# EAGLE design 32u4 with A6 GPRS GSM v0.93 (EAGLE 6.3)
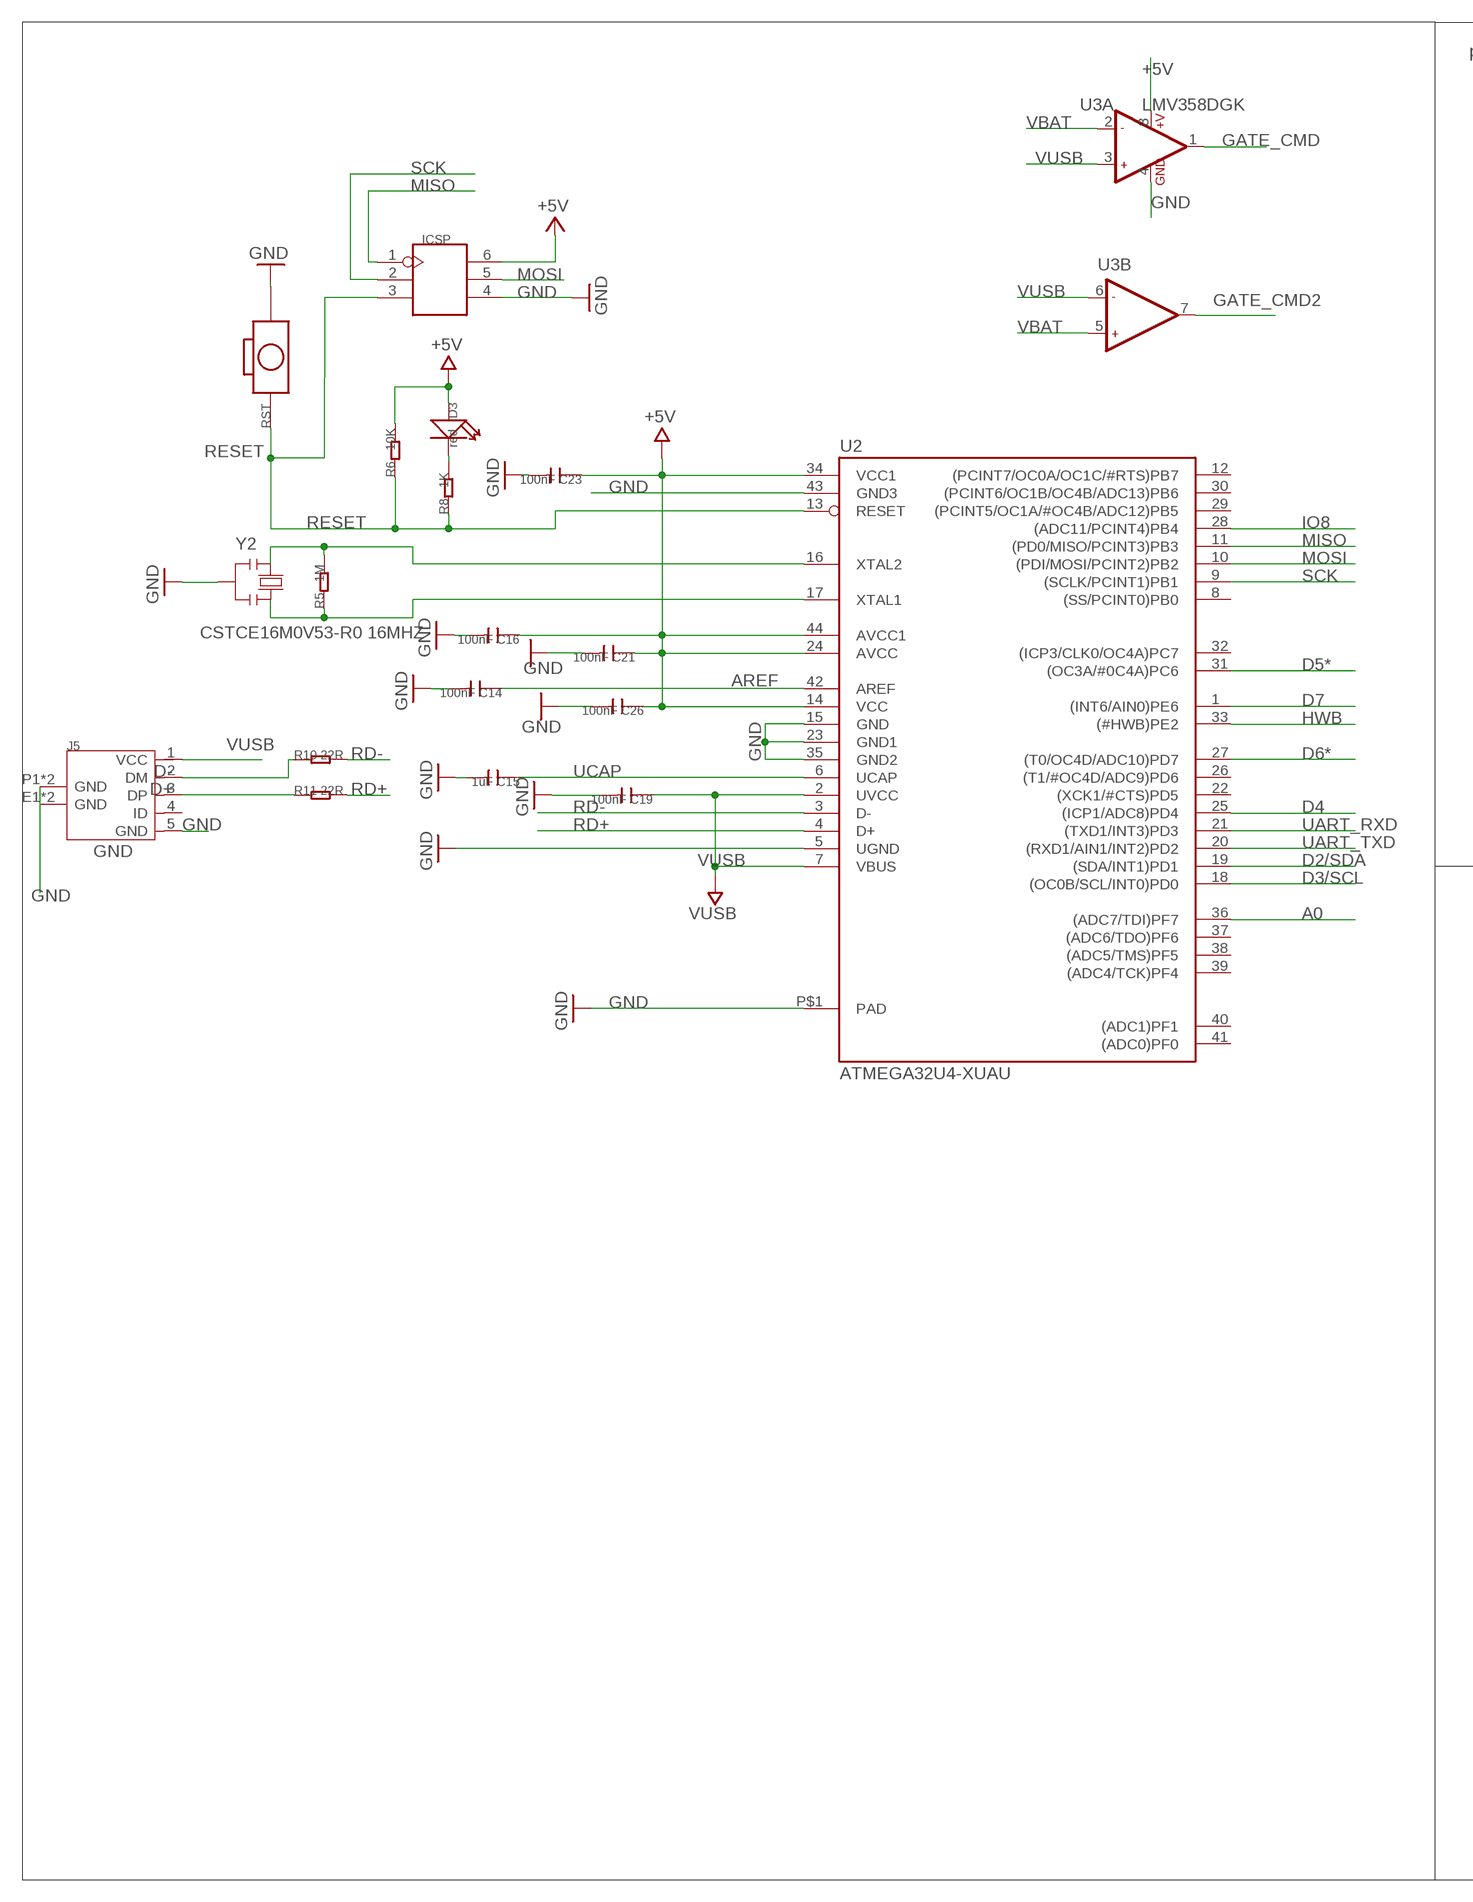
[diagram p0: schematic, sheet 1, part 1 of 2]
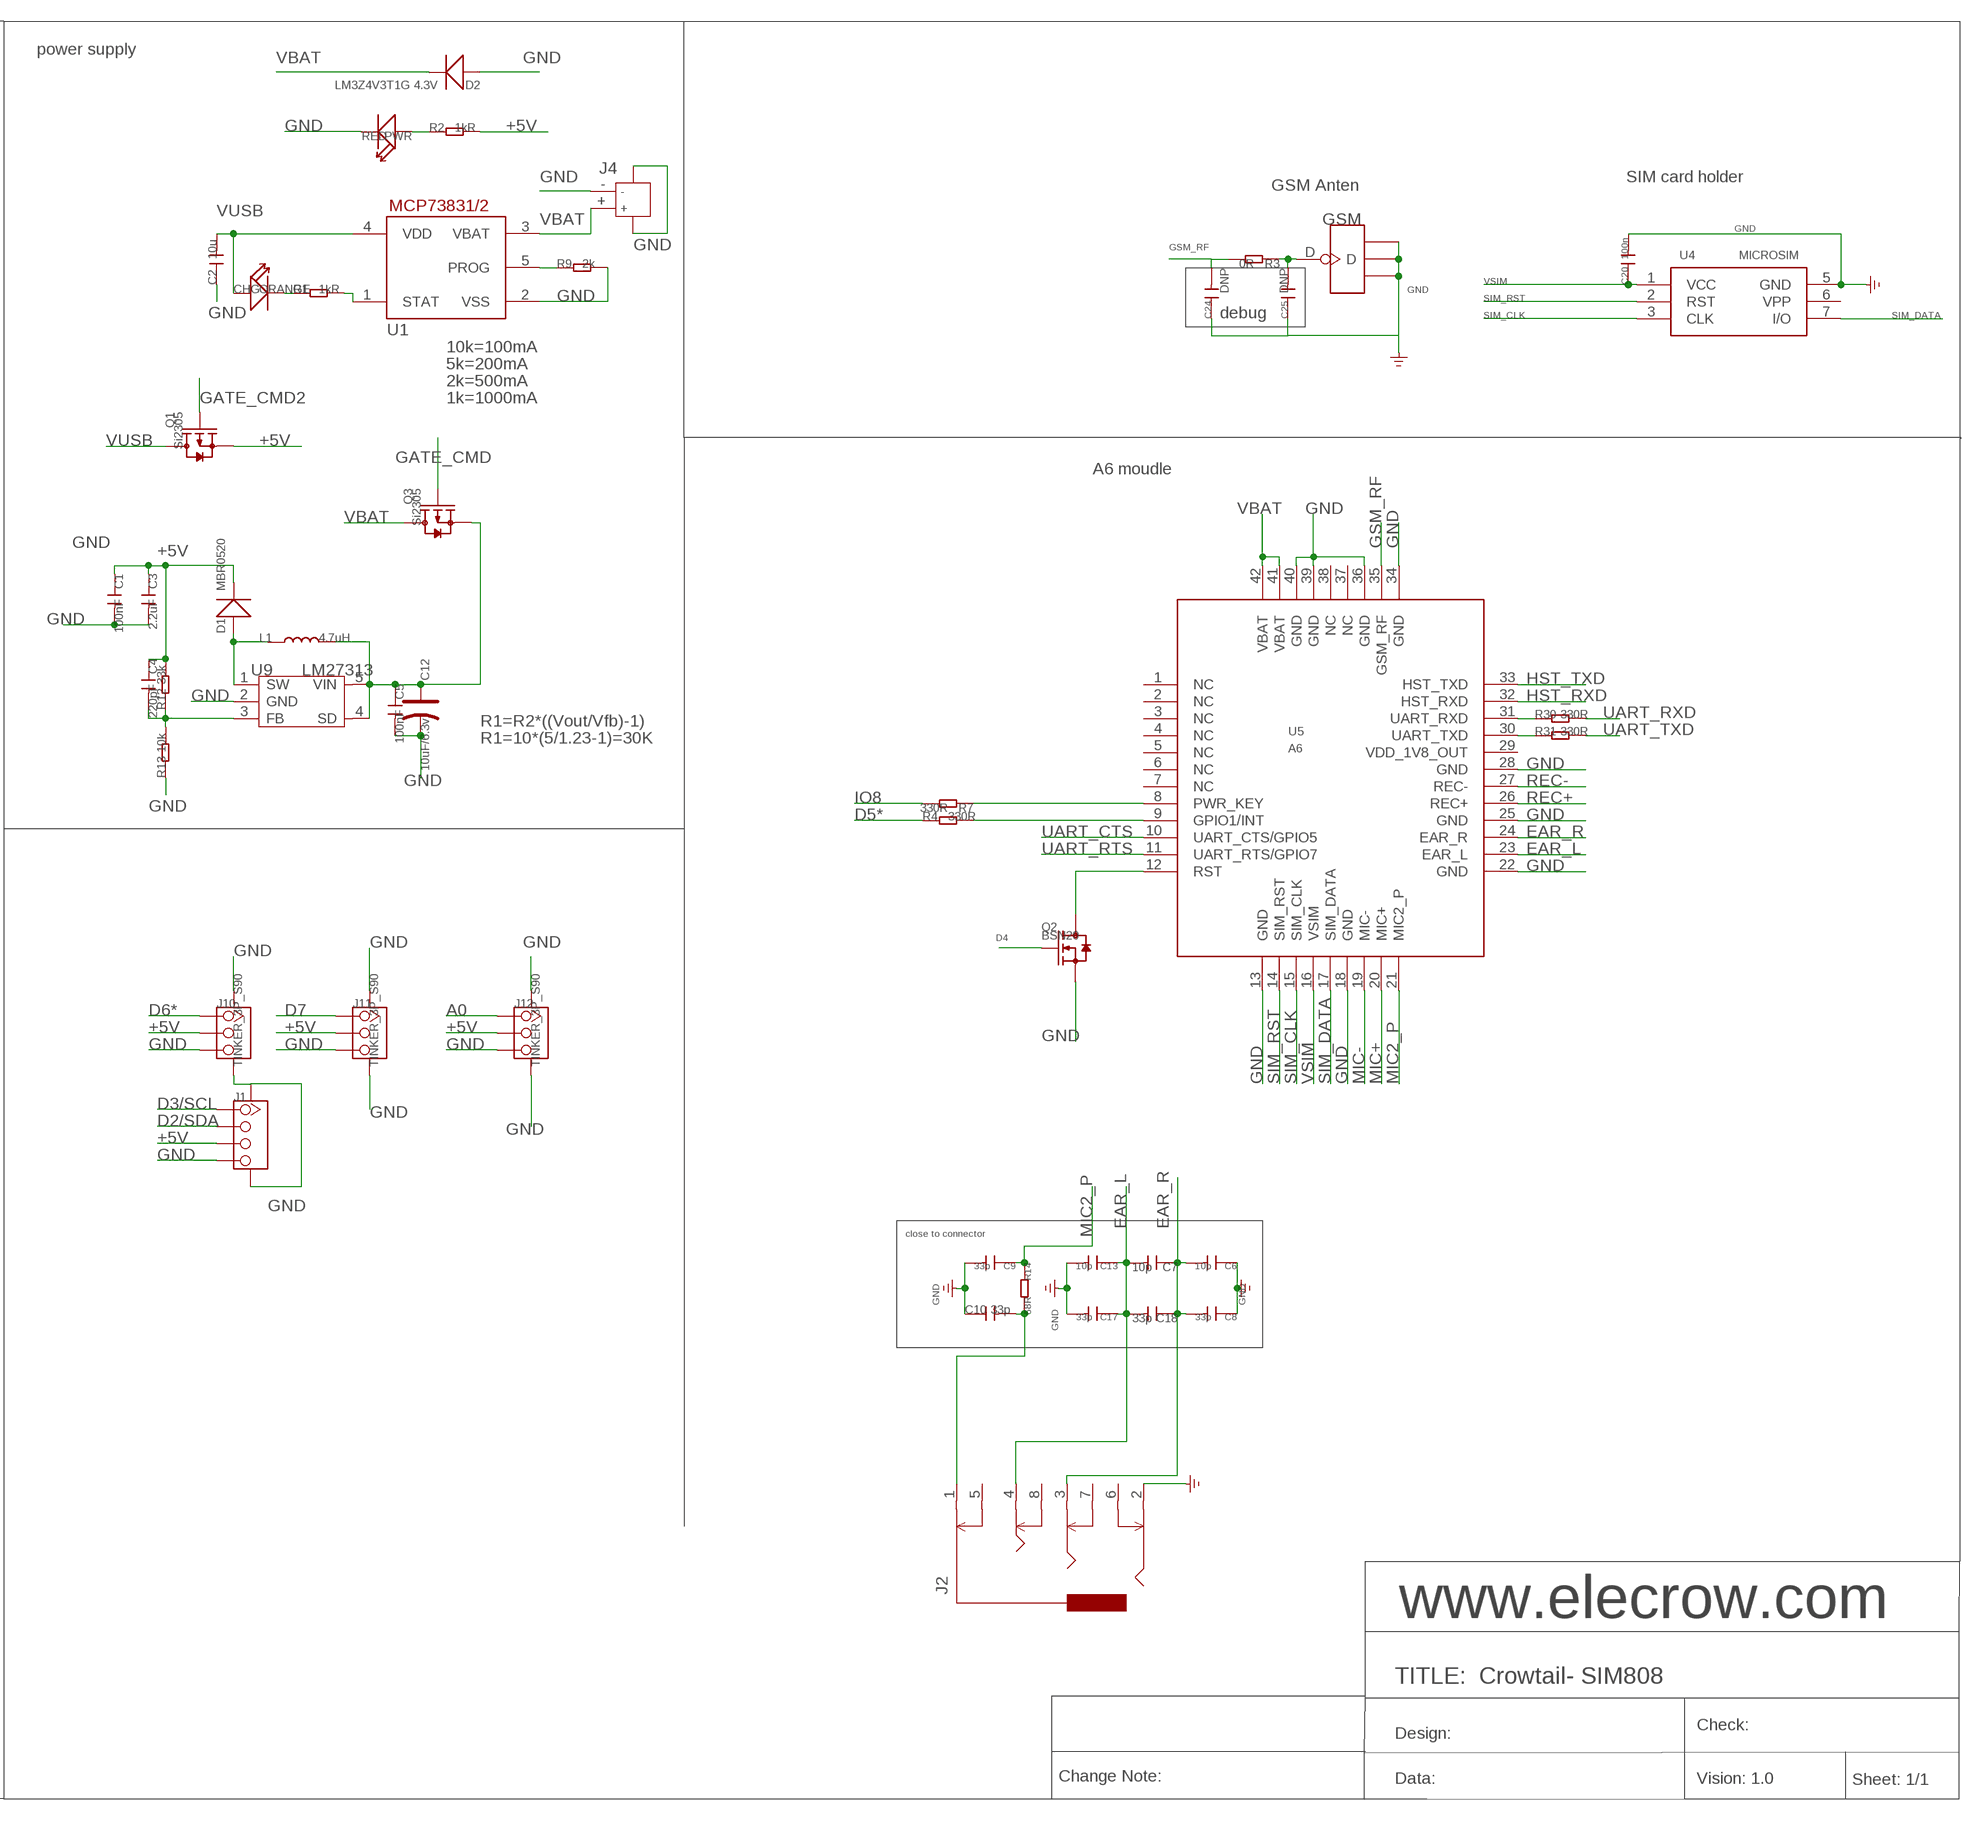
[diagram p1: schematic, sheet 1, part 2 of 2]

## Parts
C1  100nF  C-0603  [C0603]
C2  10u  C-0603  [C0603]
C3  2.2uF  C-0603  [C0603]
C4  220pF  C-0603  [C0603]
C5  100nF  C-0603  [C0603]
C6  10p  C-0402  [C0402]
C7  10p  C-0402  [C0402]
C8  33p  C-0402  [C0402]
C9  33p  C-0603  [C0603]
C10  33p  C-0603  [C0603]
C12  10uF/6.3v  CAP-AVX-A  [AVX-A]
C13  10p  C-0402  [C0402]
C14  100nF  C-0603  [C0603]
C15  1uF  C-0603  [C0603]
C16  100nF  C-0603  [C0603]
C17  33p  C-0402  [C0402]
C18  33p  C-0402  [C0402]
C19  100nF  C-0603  [C0603]
C20  100n  C-0603  [C0603]
C21  100nF  C-0603  [C0603]
C23  100nF  C-0603  [C0603]
C24  DNP  C-0402  [C0402]
C25  DNP  C-0402  [C0402]
C26  100nF  C-0603  [C0603]
CHG  ORANGE  007-LED0603  [D0603]
D1  MBR0520  D'1206'  [SOD123]
D2  LM3Z4V3T1G 4.3V  D'0805'  [SOD323]
D3  red  LED'0603'  [LED-0603]
GSM  ANTENNA-U-FL  [4P-U-FL]
ICSP  HEADER-2X3P-2.0  [2X3P-2.0]
J1  TWIG-4P-2.0-SMD-FEMALE-REINFORCE'90D'  [4P-SMD-2.0-90D]
J2  AUDIO-8P'PJ-3536-L6S'  [8P-3.5-SMD]
J4  JACK-JST-2P-SMD-PW'2.0'  [JST-SMD-2.0-90D]
J5  MICRO-USB-5P-340015001  [B-SMD-5P]
J10  TINKER_3P_S90  [TINKER_3P_S90]
J11  TINKER_3P_S90  [TINKER_3P_S90]
J12  TINKER_3P_S90  [TINKER_3P_S90]
L1  4.7uH  L  [CD32]
PWR  RED  007-LED0603  [D0603]
Q1  Si2305  MOSFET-P'SI2323CDS/SI2305DS<BR>'  [SOT23]
Q2  BSN20  MOSFET-N'SOT23'  [SOT23@1]
Q3  Si2305  MOSFET-P'SI2323CDS/SI2305DS<BR>'  [SOT23]
R1  1kR  R-0603  [R0603]
R2  1kR  R-0603  [R0603]
R3  0R  R-0603  [R0603]
R4  330R  R-0603  [R0603]
R5  1M  R-0603  [R0603]
R6  10K  R-0603  [R0603]
R7  330R  R-0603  [R0603]
R8  1K  R-0603  [R0603]
R9  2k  R-0603  [R0603]
R10  22R  R-0603  [R0603]
R11  22R  R-0603  [R0603]
R12  33k  R-0603  [R0603]
R13  10k  R-0603  [R0603]
R14  68R  R-0603  [R0603]
R30  330R  R-0603  [R0603]
R31  330R  R-0603  [R0603]
RST  BOTTON-2P-90D  [2P-7.62X3.56-90D]
U1  MCP73831/OT  [SOT23-5L]
U2  ATMEGA32U4-XUAU  [TQFP44-PAD]
U3  LMV358DGK  [MSOP8]
U4  MICROSIM  [MICROSIM]
U5  A6  [A6]
U9  LM27313  [SOT23-5]
Y2  CSTCE16M0V53-R0 16MHZ  RESONATORMU  [RESONATOR]

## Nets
+5V: C1.1 C3.1 C4.1 C16.1 C21.1 C23.1 C26.1 D1.- D3.+ ICSP.6 J1.3 J10.2 J11.2 J12.2 Q1.2(S) R2.2 R6.2 R12.2 U2.14(VCC) U2.24(AVCC) U2.34(VCC1) U2.44(AVCC1) U3.8(A:+V)
A0: J12.1 U2.36((ADC7/TDI)PF7)
AREF [aref]: C14.1 U2.42(AREF)
D2/SDA: J1.2 U2.19((SDA/INT1)PD1)
D3/SCL: J1.1 U2.18((OC0B/SCL/INT0)PD0)
D4: Q2.1(G) U2.25((ICP1/ADC8)PD4)
D5*: R4.1 U2.31((OC3A/#0C4A)PC6)
D6*: J10.1 U2.27((T0/OC4D/ADC10)PD7)
D7: J11.1 U2.1((INT6/AIN0)PE6)
D+: J5.3(DP) R11.1
D-: J5.2(DM) R10.1
EAR_L: C7.2 C13.1 C17.1 C18.2 J2.4 U5.23(EAR_L)
EAR_R: C6.2 C7.1 C8.2 C18.1 J2.3 U5.24(EAR_R)
GATE_CMD: Q3.1(G) U3.1(A:OUT1)
GATE_CMD2: Q1.1(G) U3.7(B:OUT2)
GND: C1.2 C2.1 C3.2 C5.2 C6.1 C8.1 C9.2 C10.1 C12.- C13.2 C14.2 C15.2 C16.2 C17.2 C19.2 C20.2 C21.2 C23.2 C24.1 C25.1 C26.2 D2.+ GSM.GND1 GSM.GND2 GSM.GND3 ICSP.4 J1.4 J1.SS1 J1.SS2 J2.2 J4.3 J4.4 J4.- J5.5(GND) J5.E1(GND) J5.E2(GND) J5.P1(GND) J5.P2(GND) J10.3 J10.SS1 J10.SS2 J11.3 J11.SS1 J11.SS2 J12.3 J12.SS1 J12.SS2 PWR.- Q2.2(S) R9.2 R13.1 RST.P$2 U1.2(VSS) U2.5(UGND) U2.15(GND) U2.23(GND1) U2.35(GND2) U2.43(GND3) U2.P$1(PAD) U3.4(A:GND) U4.5(GND) U5.13(GND) U5.18(GND) U5.22(GND) U5.25(GND) U5.28(GND) U5.34(GND) U5.36(GND) U5.39(GND) U5.40(GND) U9.2(GND) Y2.2
GSM_RF: C24.2 R3.2 U5.35(GSM_RF)
HST_RXD: U5.32(HST_RXD)
HST_TXD: U5.33(HST_TXD)
HWB: U2.33((#HWB)PE2)
IO8: R7.2 U2.28((ADC11/PCINT4)PB4)
MIC2_P: C9.1 R14.1 U5.21(MIC2_P)
MIC+: U5.20(MIC+)
MIC-: U5.19(MIC-)
MISO: ICSP.1 U2.11((PD0/MISO/PCINT3)PB3)
MOSI: ICSP.5 U2.10((PDI/MOSI/PCINT2)PB2)
N$5: C25.2 GSM.D R3.1
N$6: PWR.+ R2.1
N$7: R30.1 U5.31(UART_RXD)
N$8: R31.1 U5.30(UART_TXD)
N$9: R7.1 U5.8(PWR_KEY)
N$11: CHG.- R1.1
N$12: Q2.3(D) U5.12(RST)
N$13: R4.2 U5.9(GPIO1/INT)
N$14: D1.+ L1.1 U9.1(SW)
N$15: D3.- R8.2
N$16: C4.2 R12.1 R13.2 U9.3(FB)
N$20: R1.2 U1.1(STAT)
N$30: C10.2 J2.1 R14.2
N$31: R9.1 U1.5(PROG)
RD+: R11.2 U2.4(D+)
RD-: R10.2 U2.3(D-)
REC+: U5.26(REC+)
REC-: U5.27(REC-)
RESET: ICSP.3 R6.1 R8.1 RST.P$1 U2.13(RESET)
SCK: ICSP.2 U2.9((SCLK/PCINT1)PB1)
SIM_CLK: U4.3(CLK) U5.15(SIM_CLK)
SIM_DATA: U4.7(I/O) U5.17(SIM_DATA)
SIM_RST: U4.2(RST) U5.14(SIM_RST)
UART_CTS: U5.10(UART_CTS/GPIO5)
UART_RTS: U5.11(UART_RTS/GPIO7)
UART_RXD: R30.2 U2.21((TXD1/INT3)PD3)
UART_TXD: R31.2 U2.20((RXD1/AIN1/INT2)PD2)
UCAP: C15.1 U2.6(UCAP)
VBAT: D2.- J4.+ Q3.3(D) U1.3(VBAT) U3.2(A:-IN1) U3.5(B:+IN2) U5.41(VBAT) U5.42(VBAT)
VBAT1: C5.1 C12.+ L1.2 Q3.2(S) U9.4(SD) U9.5(VIN)
VSIM: C20.1 U4.1(VCC) U5.16(VSIM)
VUSB: C2.2 C19.1 CHG.+ J5.1(VCC) Q1.3(D) U1.4(VDD) U2.2(UVCC) U2.7(VBUS) U3.3(A:+IN1) U3.6(B:-IN2)
XTAL3: R5.2 U2.16(XTAL2) Y2.1
XTAL4: R5.1 U2.17(XTAL1) Y2.3
Unconnected: J2.5 J2.6 J2.7 J2.8 J5.4(ID) U2.8((SS/PCINT0)PB0) U2.12((PCINT7/OC0A/OC1C/#RTS)PB7) U2.22((XCK1/#CTS)PD5) U2.26((T1/#OC4D/ADC9)PD6) U2.29((PCINT5/OC1A/#OC4B/ADC12)PB5) U2.30((PCINT6/OC1B/OC4B/ADC13)PB6) U2.32((ICP3/CLK0/OC4A)PC7) U2.37((ADC6/TDO)PF6) U2.38((ADC5/TMS)PF5) U2.39((ADC4/TCK)PF4) U2.40((ADC1)PF1) U2.41((ADC0)PF0) U4.6(VPP) U5.1(NC) U5.2(NC) U5.3(NC) U5.4(NC) U5.5(NC) U5.6(NC) U5.7(NC) U5.29(VDD_1V8_OUT) U5.37(NC) U5.38(NC)

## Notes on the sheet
- power supply
- SIM card holder
- GSM Anten
- debug
- 10k=100mA
- 5k=200mA
- 2k=500mA
- 1k=1000mA
- A6 moudle
- R1=R2*((Vout/Vfb)-1)
- R1=10*(5/1.23-1)=30K
- close to connector
- www.elecrow.com
- TITLE:  Crowtail- SIM808
- Check:
- Design:
- Change Note: | Data: | Vision: 1.0 | Sheet: 1/1

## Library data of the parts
C1-C10 C13-C21 C23-C26 = Discrete:C*: Ceramic Capacitors
C12 = Discrete:CAP*: Electrolytic Capacitors,Tantalum Capacitors and Super Capacitors
CHG PWR = Discrete:007-LED*
D1 D2 = Discrete:D*
D3 = Discrete:LED*
GSM = Connector:ANTENNA-U-FL
ICSP = Connector:HEADER-2X3P
J1 = Connector:TWIG-4P-2.0-SMD-FEMALE-REINFORCE
J2 = template:AUDIO-8P
J4 = Connector:JACK-JST-2P-SMD-PW
J5 = OPL Eagle Library:MICRO-USB-5P: ST-USB-001E：MICRO USB B SMD R/A
J10-J12 = Connector:TINKER_3P_S90
L1 = Discrete:L*
Q1 Q3 = Discrete:MOSFET-P
Q2 = Discrete:MOSFET-N: IRLL014: http://www.vishay.com/docs/91319/sihll014.pdf
R1-R14 R30 R31 = Discrete:R*
RST = Discrete:BOTTON-2P
U1 = adafruit:MCP73831: MCP73831/2 Miniature Single-Cell, Fully Integrated Li-Ion, Li-Polymer Charge Management Controllers. Nice and small simple lipoly charge controller, with adjustable current and status output (LED) http://www.ladyada.net/library/pcb/eaglelibrary.html
U2 = SmartPrj:ATMEGA32U4-XU
U3 = IC:LMV358: General purpose LOW Voltage, Rail-to-Rail Output Amplifiers http://www.fairchildsemi.com/ds/LM/LMV358.pdf
U4 = Connector:MICROSIM
U5 = IC:A6
U9 = IC:LM27313
Y2 = SmartPrj:RESONATOR

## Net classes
0 default: width 0.203 mm, drill 0.305 mm, clearance 0.152 mm
2 gnd: width 0.305 mm, drill 0.559 mm, clearance 0.254 mm
3 usbvcc: width 0.508 mm, drill 0.61 mm, clearance 0.254 mm
4 aref: width 0.254 mm, drill 0.61 mm, clearance 0.254 mm

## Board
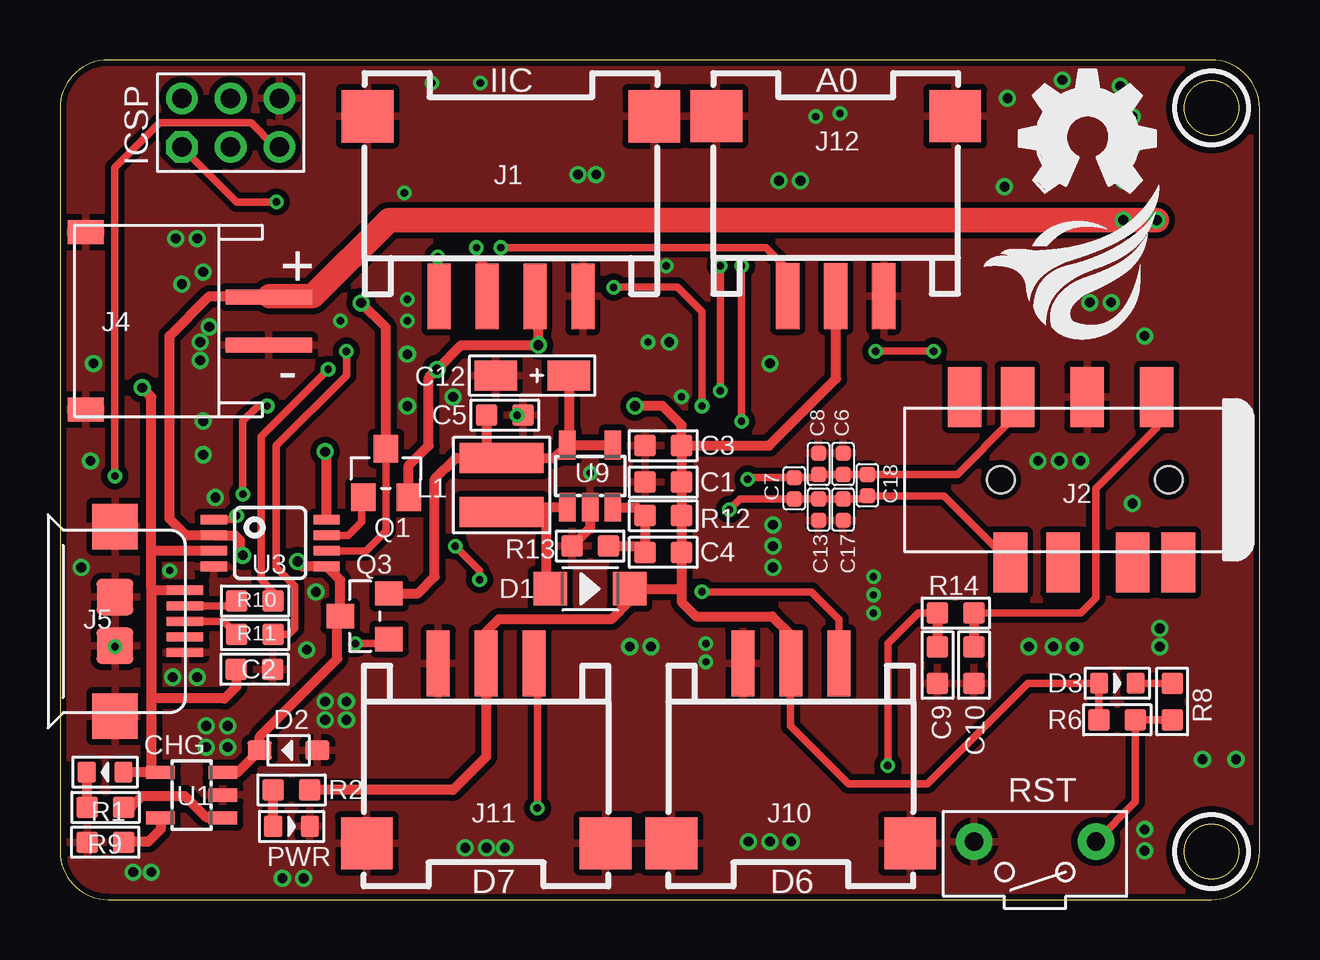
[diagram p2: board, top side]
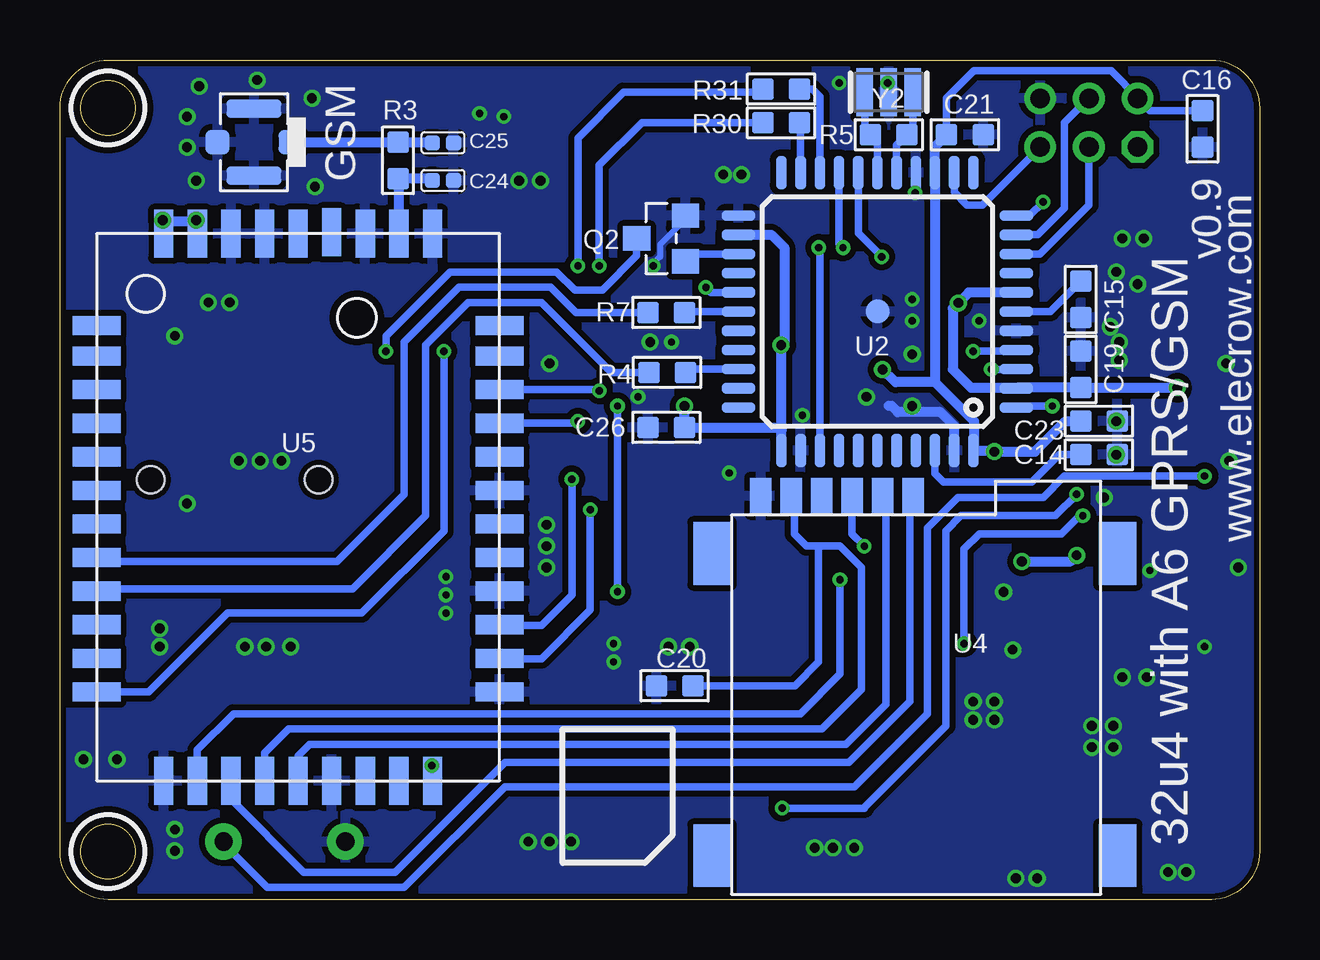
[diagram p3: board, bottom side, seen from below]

Size 50 x 35 mm. Coordinates in mm from the lower left corner, seen from the top.
Outline: 0,33 0,2 arc90 2,0 48,0 arc90 50,2 50,33 arc90 48,35 2,35 arc90 0,33
Outline: circle at 48,2 radius 1.14
Outline: circle at 48,33 radius 1.14
Copper layers (1*16): Top 0.035mm / dielectric 1.5mm / Bottom 0.035mm
Design rules "SeeedStudio_rule_no_angle_090911": minimum track width 6mil, minimum drill 12mil, track to track 6mil, track to pad 6mil, pad to pad 6mil, via to via 6mil, smd to smd 0mil, copper to edge 10mil, drill to drill 10mil, minimum pad ring 10mil, minimum via ring 6mil, stop-mask expansion 2mil, vias tented up to drill 100mil, thermal gap 10mil
tRestrict: area 35.6,41.9 to 35.7,43.3; area 46.5,0.5 to 49.5,3.5; area 46.5,31.5 to 49.5,34.5
bRestrict: area 46.5,0.5 to 49.5,3.5; area 46.5,31.5 to 49.5,34.5

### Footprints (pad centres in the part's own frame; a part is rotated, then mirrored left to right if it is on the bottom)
C0603 = smd 0.889 x 0.889: 1 -0.762,0; 2 0.762,0
C0402 = smd 0.635 x 0.635: 1 -0.445,0; 2 0.445,0
AVX-A = smd 1.778 x 1.27: + -1.524,0; - 1.524,0
D0603 = smd 0.762 x 0.889: + -0.762,0; - 0.762,0
SOD123 = smd 1.397 x 1.397: + -1.651,0; - 1.651,0
SOD323 = smd 1 x 0.8: + -1.2,0; - 1.2,0
LED-0603 = smd 0.762 x 0.889: + -0.762,0; - 0.762,0
4P-U-FL = smd 1.016 x 1.016: D -1.524,0; GND3 1.524,0 | smd 2.286 x 0.762: GND1 0,1.397; GND2 0,-1.397
2X3P-2.0 = drill 0.813 pad 1.27 octagon: 1 -1.016,2.032 | drill 0.813 pad 1.27: 2 -1.016,0; 3 -1.016,-2.032; 4 1.016,-2.032; 5 1.016,0; 6 1.016,2.032
4P-SMD-2.0-90D = smd 0.965 x 2.74: 1 -3,-0.1; 2 -1,-0.1; 3 1,-0.1; 4 3,-0.1 | smd 2.159 x 2.184: SS1 -5.974,7.4; SS2 5.974,7.4
8P-3.5-SMD = smd 1.4 x 2.5: 1 2.8,-3.45; 2 5.7,-3.45; 3 8.6,-3.45; 4 8.9,3.45; 5 1.9,3.45; 6 3.8,3.45; 7 6.7,3.45; 8 10.8,-3.45 | hole 1.149: 2.3,0; 9.3,0
JST-SMD-2.0-90D = smd 1 x 1.5: 3 3.7,-2.54; 4 -3.7,-2.54 | smd 0.635 x 3.6: + -1,5.08; - 1,5.08
B-SMD-5P = smd 0.38 x 1.52: 1 -1.3,2.54; 2 -0.65,2.54; 3 0,2.54; 4 0.65,2.54; 5 1.3,2.54 | smd 1.524 x 1.524: E1 -1.016,-0.381; E2 1.016,-0.381 | smd 1.9 x 1.9: P1 -3.95,-0.381; P2 3.95,-0.381
TINKER_3P_S90 = smd 0.965 x 2.74: 1 -1.984,-4.545; 2 0.016,-4.545; 3 2.016,-4.545 | smd 2.159 x 2.184: SS1 -4.958,2.955; SS2 4.99,2.955
CD32 = smd 3.5 x 1.25: 1 0,1.125; 2 0,-1.125
SOT23 = smd 1.016 x 1.143: 1 -0.95,-1.016; 2 0.95,-1.016; 3 0,1.016
SOT23@1 = smd 1.016 x 1.143: 1 -0.95,-1.016; 2 0.95,-1.016; 3 0,1.016
R0603 = smd 0.889 x 0.889: 1 -0.762,0; 2 0.762,0
2P-7.62X3.56-90D = drill 0.762 pad 1.524: P$1 0,2.54; P$2 0,-2.54
SOT23-5L = smd 0.55 x 1.2: 1 -0.95,-1.3; 2 0,-1.3; 3 0.95,-1.3; 4 0.95,1.3; 5 -0.95,1.3
TQFP44-PAD = smd 1.4 x 0.45: 1 -5.8,4; 2 -5.8,3.2; 3 -5.8,2.4; 4 -5.8,1.6; 5 -5.8,0.8; 6 -5.8,0; 7 -5.8,-0.8; 8 -5.8,-1.6; 9 -5.8,-2.4; 10 -5.8,-3.2; 11 -5.8,-4; 23 5.8,-4; 24 5.8,-3.2; 25 5.8,-2.4; 26 5.8,-1.6; 27 5.8,-0.8; 28 5.8,0; 29 5.8,0.8; 30 5.8,1.6; 31 5.8,2.4; 32 5.8,3.2; 33 5.8,4 | smd 0.45 x 1.4: 12 -4,-5.8; 13 -3.2,-5.8; 14 -2.4,-5.8; 15 -1.6,-5.8; 16 -0.8,-5.8; 17 0,-5.8; 18 0.8,-5.8; 19 1.6,-5.8; 20 2.4,-5.8; 21 3.2,-5.8; 22 4,-5.8; 34 4,5.8; 35 3.2,5.8; 36 2.4,5.8; 37 1.6,5.8; 38 0.8,5.8; 39 0,5.8; 40 -0.8,5.8; 41 -1.6,5.8; 42 -2.4,5.8; 43 -3.2,5.8; 44 -4,5.8 | smd 1 x 1: P$1 0,0
MSOP8 = smd 0.4 x 1.1: 1 -0.975,-2.35; 2 -0.325,-2.35; 3 0.325,-2.35; 4 0.975,-2.35; 5 0.975,2.35; 6 0.325,2.35; 7 -0.325,2.35; 8 -0.975,2.35
MICROSIM = smd 1.5 x 0.9: 1 -0.8,2.5; 2 -0.8,5.04; 3 -0.8,7.58; 5 -0.8,1.23; 6 -0.8,3.77; 7 -0.8,6.31 | smd 2.61 x 1.56: P$1 1.6,-0.8; P$2 14.2,-0.8; P$3 14.2,16.1; P$4 1.6,16.1
A6 = smd 0.8 x 2: 1 7.57,8.4; 2 6.3,8.4; 3 4.9,8.4; 4 3.5,8.4; 5 2.1,8.4; 6 0.7,8.4; 7 -0.7,8.4; 8 -2.1,8.4; 9 -3.5,8.4; 10 -4.9,8.4; 11 -6.3,8.4; 12 -7.7,8.4; 22 -7.7,-8.4; 23 -6.3,-8.4; 24 -4.9,-8.4; 25 -3.5,-8.4; 26 -2.1,-8.4; 27 -0.7,-8.4; 28 0.7,-8.4; 29 2.1,-8.4; 30 3.5,-8.4; 31 4.9,-8.4; 32 6.3,-8.4; 33 7.57,-8.4 | smd 2 x 0.8: 13 -11.4,5.6; 14 -11.4,4.2; 15 -11.4,2.8; 16 -11.4,1.4; 17 -11.4,0; 18 -11.4,-1.4; 19 -11.4,-2.8; 20 -11.4,-4.2; 21 -11.4,-5.6; 34 11.4,-5.6; 35 11.4,-4.2; 36 11.4,-2.8; 37 11.46,-1.4; 38 11.4,0; 39 11.4,1.4; 40 11.4,2.8; 41 11.4,4.2; 42 11.4,5.6
SOT23-5 = smd 0.69 x 1.2: 1 -0.95,-1.3; 2 0,-1.3; 3 0.95,-1.3; 4 0.95,1.3; 5 -0.95,1.3
RESONATOR = smd 0.7 x 2: 1 -1,0; 2 0,0; 3 1,0

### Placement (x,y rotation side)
C1  25.15,17.4 180 top
C2  8.11,9.6 180 top
C3  25.15,18.92 180 top
C4  25.15,14.48 180 top
C5  18.54,20.19 0 top
C6  32.64,18.16 270 top
C7  30.61,17.14 270 top
C8  31.62,18.16 270 top
C9  36.58,9.78 270 top
C10  38.1,9.78 90 top
C12  19.68,21.84 180 top
C13  31.62,16.26 270 top
C14  6.69,18.54 0 bottom
C15  7.46,25.02 270 bottom
C16  2.38,32.13 270 bottom
C17  32.64,16.26 270 top
C18  33.66,17.27 270 top
C19  7.46,22.1 90 bottom
C20  24.38,8.91 180 bottom
C21  12.28,31.88 0 bottom
C23  6.69,19.94 0 bottom
C24  34.04,29.97 180 bottom
C25  34.04,31.55 180 bottom
C26  24.73,19.68 180 bottom
CHG  1.88,5.31 180 top
D1  22.1,12.95 0 top
D2  9.53,6.22 180 top
D3  44.07,9.02 0 top
GSM  41.91,31.57 180 bottom
ICSP  7.11,32.38 90 top
J1  18.8,25.25 0 top
J2  48.51,17.5 180 top
J4  3.62,24.12 270 top
J5  2.67,11.6 270 top
J10  30.48,5.3 180 top
J11  17.78,5.3 180 top
J12  32.32,29.7 0 top
L1  18.41,17.27 180 top
LOGO2  LOGO-OSHW-FILLX0200-NT  [OSHW_FILLX200_NOTEXT]  39.99,29.5 0 top
PWR  9.65,3.05 0 top
Q1  13.59,17.78 0 top
Q2  24.94,27.56 90 bottom
Q3  12.7,11.81 90 top
R1  1.9,3.84 0 top
R2  9.65,4.57 0 top
R3  35.91,30.82 270 bottom
R4  24.69,21.97 180 bottom
R5  15.46,31.88 0 bottom
R6  44.07,7.49 180 top
R7  24.73,24.47 0 bottom
R8  46.35,8.26 90 top
R9  1.89,2.39 180 top
R10  8.13,12.45 0 top
R11  8.13,11.05 0 top
R12  25.15,16 0 top
R13  22.1,14.73 0 top
R14  37.34,11.94 0 top
R30  19.94,32.38 0 bottom
R31  19.94,33.78 0 bottom
RST  40.64,2.41 270 top
U1  5.49,4.36 90 top
U2  15.93,24.51 180 bottom
U3  8.76,14.86 270 top
U4  22.01,16.03 270 bottom
U5  40.08,16.36 90 bottom
U9  22.1,17.65 0 top
U$4  [ELECROW_NRW_6]  38.5,23.35 0 top
Y2  15.46,33.66 180 bottom

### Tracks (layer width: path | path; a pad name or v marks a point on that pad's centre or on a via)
+5V  (via drill 0.41)
  Top 0.305: R6.2 D3.+ 40.35,9.02 36.16,4.83 32.85,4.83 30.44,7.24 30.44,9.82 J10.2
  Top 0.406: C3.1 C1.1 R12.2 C4.1 25.91,12.95 | C3.1 25.91,19.77 25.11,20.57 v23.96,20.57 | C3.1 29.55,18.92 32.35,21.72 32.35,25.14 J12.2 | 25.91,12.95 25.91,12.41 26.5,11.81 29.68,11.81 30.44,11.05 30.44,9.91 30.57,9.78 30.53,9.78 J10.2 | 25.91,12.95 D1.- 23.75,12.45 22.99,11.68 18.29,11.68 17.76,11.16 J11.2 17.76,5.95 16.38,4.57 R2.2 | U3.8 11.11,18.61 v11.05,18.67 | Q1.2 14.54,18.09 15.37,18.92 15.37,21.75 v15.71,22.1 16.73,23.11 v19.94,23.11 19.94,25.01 J1.3
  Bottom 0.305: C16.1 4.57,32.89 ICSP.6 5.04,33.4 6.18,34.54 11.9,34.54 13.04,33.4 C21.1
  Bottom 0.406: U2.34 19.93,19.56 | C21.1 13.53,31.39 U2.14 13.53,21.57 | v23.96,20.57 C26.1 20.05,19.68 19.93,19.56 | 13.53,21.57 11.9,19.94 11.9,18.74 U2.44 11.09,18.71 v11.05,18.67 9.36,18.67 8.09,19.94 C23.1 | 13.53,21.57 15.18,21.57 v15.71,22.1 | 19.93,19.56 19.93,23.1 v19.94,23.11 19.81,23.24 19.81,27.18 20.34,27.71 U2.24
A0  (via drill 0.3)
  Top 0.305: v18.38,27.18 29.43,27.18 30.44,26.16 30.44,25.15 30.32,25.27
  Top 0.406: 30.48,25.27 30.36,25.16 J12.1 30.34,25.15 30.44,25.15
  Bottom 0.305: U2.36 18.33,27.13 v18.38,27.18
AREF
  Bottom 0.305: C14.1 8.34,18.54 9.49,17.4 13.17,17.4 13.53,17.75 U2.42
D2/SDA  (via drill 0.3)
  Top 0.305: v17.36,27.18 17.36,26.8 17.74,26.42 17.74,25.4 18,25.15 J1.2 | 17.74,25.15 J1.2 | J1.2
  Bottom 0.305: U2.19 17.53,27.34 v17.36,27.18
D3/SCL  (via drill 0.3)
  Top 0.406: v15.75,26.8 15.75,25.2 J1.1
  Bottom 0.305: U2.18 16.73,27.77 v15.75,26.8
D4
  Bottom 0.305: U2.25 23.62,26.91 Q2.1
D5*
  Bottom 0.305: U2.31 23.79,22.11 R4.1
D6*  (via drill 0.3)
  Top 0.305: v23.08,25.53 25.74,25.53 26.76,24.51 v26.76,20.57 | v26.76,12.83 31.33,12.83 32.47,11.68 32.47,9.86 J10.1
  Bottom 0.305: U2.27 22.86,25.31 v23.08,25.53 | v26.76,20.57 v26.76,12.83
D7  (via drill 0.3)
  Top 0.305: v19.9,3.81 19.9,9.71 J11.1 | v7.62,16.89 7.62,19.94 8.26,20.57 v8.64,20.57
  Bottom 0.305: v19.9,3.81 16.47,3.81 16.47,3.85 13.08,7.24 13.08,15.37 12.45,16 8.51,16 v7.62,16.89 | v8.64,20.57 10.06,20.57 U2.1
D+
  Top 0.305: J5.3 6.82,11.6 R11.1
D-
  Top 0.305: J5.2 7.17,12.24 R10.1
EAR_L  (via drill 0.3)
  Top 0.305: v27.9,16.26 28.35,16.7 C7.2 C13.1 C17.1 33.53,16.7 C18.2 36.84,16.83 J2.4
  Bottom 0.305: v27.9,16.26 27.9,12.06 29.93,10.03 31.65,10.03 U5.23
EAR_R  (via drill 0.3)
  Top 0.305: v28.66,17.53 28.73,17.59 C7.1 31.5,17.59 C8.2 C6.2 C18.1 37.4,17.72 39.62,19.94 39.62,20.66 J2.3
  Bottom 0.305: v28.66,17.53 28.66,12.7 29.93,11.43 31.65,11.43 U5.24
GATE_CMD  (via drill 0.3)
  Top 0.305: U3.1 7.2,15.83 v7.37,16 | v12.32,10.67 13.52,10.67 Q3.1
  Bottom 0.305: v7.37,16 7.49,16 8.26,15.24 11.68,15.24 12.32,14.61 v12.32,10.67
GATE_CMD2
  Top 0.305: 12.7,16.82 Q1.1 12.57,16.7 12.57,15.75 12.01,15.18 U3.7
GND  (via drill 0.3, 0.41)
  Top 0.406: U9.2 22.1,15.49 R13.1
  Bottom 0.254: Q2.2 23.93,28.36 24.98,27.3 24.98,26.8 25.36,26.42 v25.27,26.42
  Bottom 0.406: Y2.2 15.46,34 v15.49,34.04 | U2.43 12.73,19.75 13.3,20.32 15.07,20.32 15.33,20.57 15.46,20.57 | U2.15 14.33,29.6 14.31,29.59 14.44,29.46 v14.35,29.46 14.31,29.46
  other vias: 14.48,25.02 14.48,24.13 11.68,24.13 22.1,17.78 19.05,20.19 26.92,10.67 26.92,9.91 33.91,13.46 33.91,12.7 33.91,11.94 4.57,13.72 2.29,10.54 24.51,23.24 21.59,30.23 22.35,30.23 17.53,34.04 31.5,32.64 32.51,32.77 25.91,20.95 40.39,10.54 41.4,10.54 28.7,2.41 29.59,2.41 17.78,2.16 16.89,2.16 10.16,0.89 9.27,0.89 4.7,9.27 6.1,6.35 5.08,25.65 1.27,18.29 5.71,27.56 4.83,27.56 14.48,22.73 25.4,23.24 29.59,22.35 43.81,24.89 42.93,24.89 41.66,18.29 16.38,20.95 14.48,20.57 45.85,11.3 24.64,10.54 23.75,10.54 29.72,13.84 29.97,29.97 30.86,29.97 41.78,34.16 44.2,33.91 44.7,32.64 44.7,31.37 44.32,29.97 39.37,29.72 39.5,33.4 0.89,13.84 1.4,22.35 5.71,9.27 6.99,6.35 11.94,8.26 11.05,7.49 30.48,2.41 3.05,1.14 3.81,1.14 10.67,12.83 11.05,8.26 11.94,7.49 6.48,16.76 5.84,23.24 5.84,22.48 5.97,18.54 5.97,19.94 5.97,26.16 10.29,10.41 6.99,7.24 6.1,7.24 18.54,2.16 29.72,14.73 29.72,15.62 45.85,10.54 42.29,10.54 47.62,5.84 49.02,5.84 40.77,18.29 42.55,18.29 44.7,16.51 45.21,23.5 45.21,2.92 45.21,2.03 6.22,23.88
  pour Bottom (isolate 0.254): -1.27,-1.27 50.8,-1.27 50.8,35.56 -1.27,35.56
  pour Top (isolate 0.254): -1.27,-1.27 50.8,-1.27 50.8,35.56 -1.27,35.56
GSM_RF
  Bottom 0.406: U5.35 35.88,29.97 | 35.88,29.97 35.88,30.07 | 35.88,30.07 35.9,30.1 | R3.2 35.91,30.01 35.88,29.97 | 35.88,30.07 34.48,30.07 C24.2
IO8
  Bottom 0.305: U2.28 23.93,24.51 R7.2
MIC2_P  (via drill 0.3)
  Top 0.305: v34.51,5.59 34.51,10.67 35.78,11.94 R14.1
  Top 0.406: R14.1 C9.1
  Bottom 0.305: U5.21 34.48,5.56 v34.51,5.59
MISO  (via drill 0.3)
  Top 0.305: v9.02,29.08 7.37,29.08 ICSP.1
  Bottom 0.305: U2.11 9.59,28.51 v9.02,29.08
MOSI
  Bottom 0.305: U2.10 9.25,27.71 8.13,28.83 8.13,32.38 ICSP.5
N$5
  Bottom 0.406: GSM.D 35.98,31.57 35.91,31.5 | C25.2 35.83,31.55 35.9,31.62 35.9,31.5 | 35.91,31.5 R3.1 36.11,31.58 36.16,31.62 35.78,31.62 | 35.91,31.5 35.9,31.5 | 35.9,31.5 35.78,31.62 | 35.65,31.62 35.78,31.62
N$6
  Top 0.406: PWR.+ R2.1
N$7  (via drill 0.3)
  Top 0.305: v27.52,21.21 v27.52,26.42
  Bottom 0.305: 20.66,32.38 R30.1 25.74,32.38 27.52,30.61 v27.52,26.42 | U5.31 27.57,21.26 v27.52,21.21
N$8  (via drill 0.3)
  Top 0.305: v28.41,19.94 v28.41,26.42
  Bottom 0.305: U5.30 28.49,19.86 v28.41,19.94 | v28.41,26.42 28.41,31.75 26.5,33.66 20.83,33.66 R31.1
N$9
  Bottom 0.305: R7.1 28.5,24.47 29.55,25.53 33.36,25.53 35.65,23.24 35.65,16.89 38.44,14.1 48.31,14.1 U5.8
N$11
  Top 0.406: CHG.- 1.12,3.86 R1.1
N$12  (via drill 0.3)
  Top 0.305: v34,22.86 v36.41,22.86
  Bottom 0.305: U5.12 46.3,8.66 43.02,11.94 37.43,11.94 34,15.37 v34,22.86 | v36.41,22.86 36.41,23.5 33.74,26.16 29.3,26.16 28.54,25.4 27.39,25.4 25.96,26.84 Q2.3
N$13
  Bottom 0.305: R4.2 27.01,21.97 29.93,24.89 32.98,24.89 34.76,23.11 34.76,16 37.81,12.95 48.38,12.95 U5.9
N$14
  Top 0.406: U9.1 20.03,16.35 | 20.03,16.35 18.6,16.35 18.39,16.15 | L1.1 18.39,16.15 | 18.39,16.15 18.38,16.13 | D1.+ 20.45,13.3 20.28,13.46 20.28,16.1 20.03,16.35
N$15
  Top 0.305: R8.2 D3.-
N$16
  Top 0.406: U9.3 24.03,16.35 R12.1 C4.2 24.26,14.35 24.26,14.61 24.13,14.73 R13.2
N$20
  Top 0.406: R1.2 2.95,3.84 3.43,4.32 5.21,4.32 6.1,3.43 6.77,3.43 U1.1
N$30
  Top 0.305: R14.2 42.55,11.94 43.18,12.57 43.18,17.14 45.72,19.68 J2.1
  Top 0.406: R14.2 C10.2
N$31
  Top 0.406: U1.5 4.19,2.92 3.68,2.41 2.68,2.41 R9.1
RD+  (via drill 0.3)
  Top 0.305: R11.2 9.53,11.05 9.78,11.3 9.78,13.08 9.02,13.84 9.02,18.92 11.94,21.84 v11.94,22.86
  Bottom 0.305: v11.94,22.86 10.18,22.86 U2.4
RD-  (via drill 0.3)
  Top 0.305: R10.2 8.89,12.83 8.38,13.34 8.38,19.3 v11.18,22.1
  Bottom 0.305: v11.18,22.1 10.14,22.1 U2.3
RESET  (via drill 0.3)
  Top 0.305: R8.1 R6.1 44.83,4.06 RST.P$1 | ICSP.3 8.98,31.37 7.96,32.38 4.15,32.38 2.29,30.52 v2.29,17.65
  Bottom 0.305: U2.13 12.73,29.49 12.19,28.96 11.56,28.96 ICSP.3 | RST.P$1 43.27,2.41 41.36,0.51 35.65,0.51 31.46,4.7 16.89,4.7 13.84,7.75 13.84,15.49 12.57,16.76 9.02,16.76 8.13,17.65 v2.29,17.65
SCK
  Bottom 0.305: U2.9 9.16,26.91 7.11,28.96 ICSP.2
SIM_CLK
  Bottom 0.305: U5.15 42.88,4.18 39.84,1.14 36.03,1.14 31.46,5.71 17.11,5.71 14.57,8.26 14.57,16.7 U4.3
SIM_DATA
  Bottom 0.305: U5.17 40.08,5.99 39.59,6.48 17.23,6.48 15.58,8.13 15.58,16.71 U4.7
SIM_RST  (via drill 0.3)
  Top 0.305: v17.49,13.34 17.49,13.72 v16.47,14.73
  Bottom 0.305: U5.14 44.27,6.23 42.76,7.75 19.14,7.75 17.49,9.4 v17.49,13.34 | v16.47,14.73 16.98,15.24 16.98,16.76 | 16.98,16.89 16.98,16.76 | U4.2 16.97,16.77 16.98,16.76
UART_RXD
  Bottom 0.305: U2.21 19.13,32.33 R30.2
UART_TXD
  Bottom 0.305: U2.20 18.33,33.48 18.63,33.78 R31.2
UCAP
  Bottom 0.305: U2.6 8.72,24.51 C15.1
VBAT  (via drill 0.41)
  Top 0.406: 8.73,25.15 J4.+ | 13.72,28.32 13.72,28.07 13.46,27.81 | 8.6,25.02 J4.+ | v7.62,14.35 7.49,14.48 7.49,14.99 7.29,15.18 U3.2 5.26,15.18 4.57,15.88 4.57,23.5 6.22,25.15 8.67,25.15 J4.+ | v9.91,14.1 10.12,13.88 U3.5 11.68,13.31 Q3.3 11.56,11.68 11.56,10.03 8.32,6.8 D2.- 7.41,5.31 U1.3
  Top 1.016: 8.73,25.15 10.54,25.15 13.72,28.32 v45.72,28.32
  Bottom 0.406: U5.41 44.27,28.27 v44.32,28.32 44.37,28.28 45.67,28.28 | U5.42 45.67,28.28 | 45.67,28.28 v45.72,28.32 | v9.91,14.1 7.87,14.1 v7.62,14.35
VBAT1
  Top 0.406: C12.+ 21.21,19.01 U9.5 | L1.2 20.59,18.4 U9.5 | U9.5 U9.4 | Q3.2 14.92,12.76 15.62,13.46 15.62,17.53 16.51,18.41 18.4,18.41 L1.2 | C5.1 17.78,18.54 18.27,18.54 L1.2
VSIM
  Bottom 0.305: U5.16 41.48,6.11 40.48,7.11 18.25,7.11 16.6,8.76 16.6,13.84 17.49,14.73 18.38,14.73 | 19.27,16.58 U4.1 19.39,16.95 | 18.38,14.73 18.89,14.73 19.39,15.24 19.39,16.95 | C20.1 19.37,8.91 18.38,9.91 18.38,14.73 | 19.39,17.02 19.39,16.95
VUSB  (via drill 0.41)
  Top 0.305: U3.6 12.76,14.53 13.59,15.37 Q1.3
  Top 0.406: 4.26,12.89 J5.1 3.87,12.89 3.81,12.95 | 3.81,12.95 3.81,8.38 | 3.81,8.38 3.81,5.43 3.68,5.31 | U1.4 3.68,5.31 | 3.68,5.31 CHG.+ | U3.3 3.87,14.53 3.81,14.48 | Q1.3 13.59,23.84 v12.55,24.87 | C2.2 7.34,8.87 6.86,8.38 3.81,8.38 | 3.81,12.95 3.81,14.48 | 3.81,14.48 3.81,20.95 v3.43,21.34
  Bottom 0.305: 10.1,21.34 U2.2 10.15,21.34
  Bottom 0.406: 10.1,21.34 C19.1 v3.43,21.34 | U2.7 12.12,25.31 v12.55,24.87 | v12.55,24.87 12.79,24.64 12.79,22.1 12.03,21.34 10.15,21.34 | v12.55,24.87 12.55,25
XTAL3
  Bottom 0.305: U2.16 15.13,31.45 R5.2 14.46,32.12 Y2.1
XTAL4
  Bottom 0.305: U2.17 15.93,31.59 R5.1 16.46,32.12 Y2.3

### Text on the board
tPlace: IIC | A0 | + | - | D7 | D6
bPlace: v0.9 | www.elecrow.com | 32u4 with A6 GPRS/GSM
